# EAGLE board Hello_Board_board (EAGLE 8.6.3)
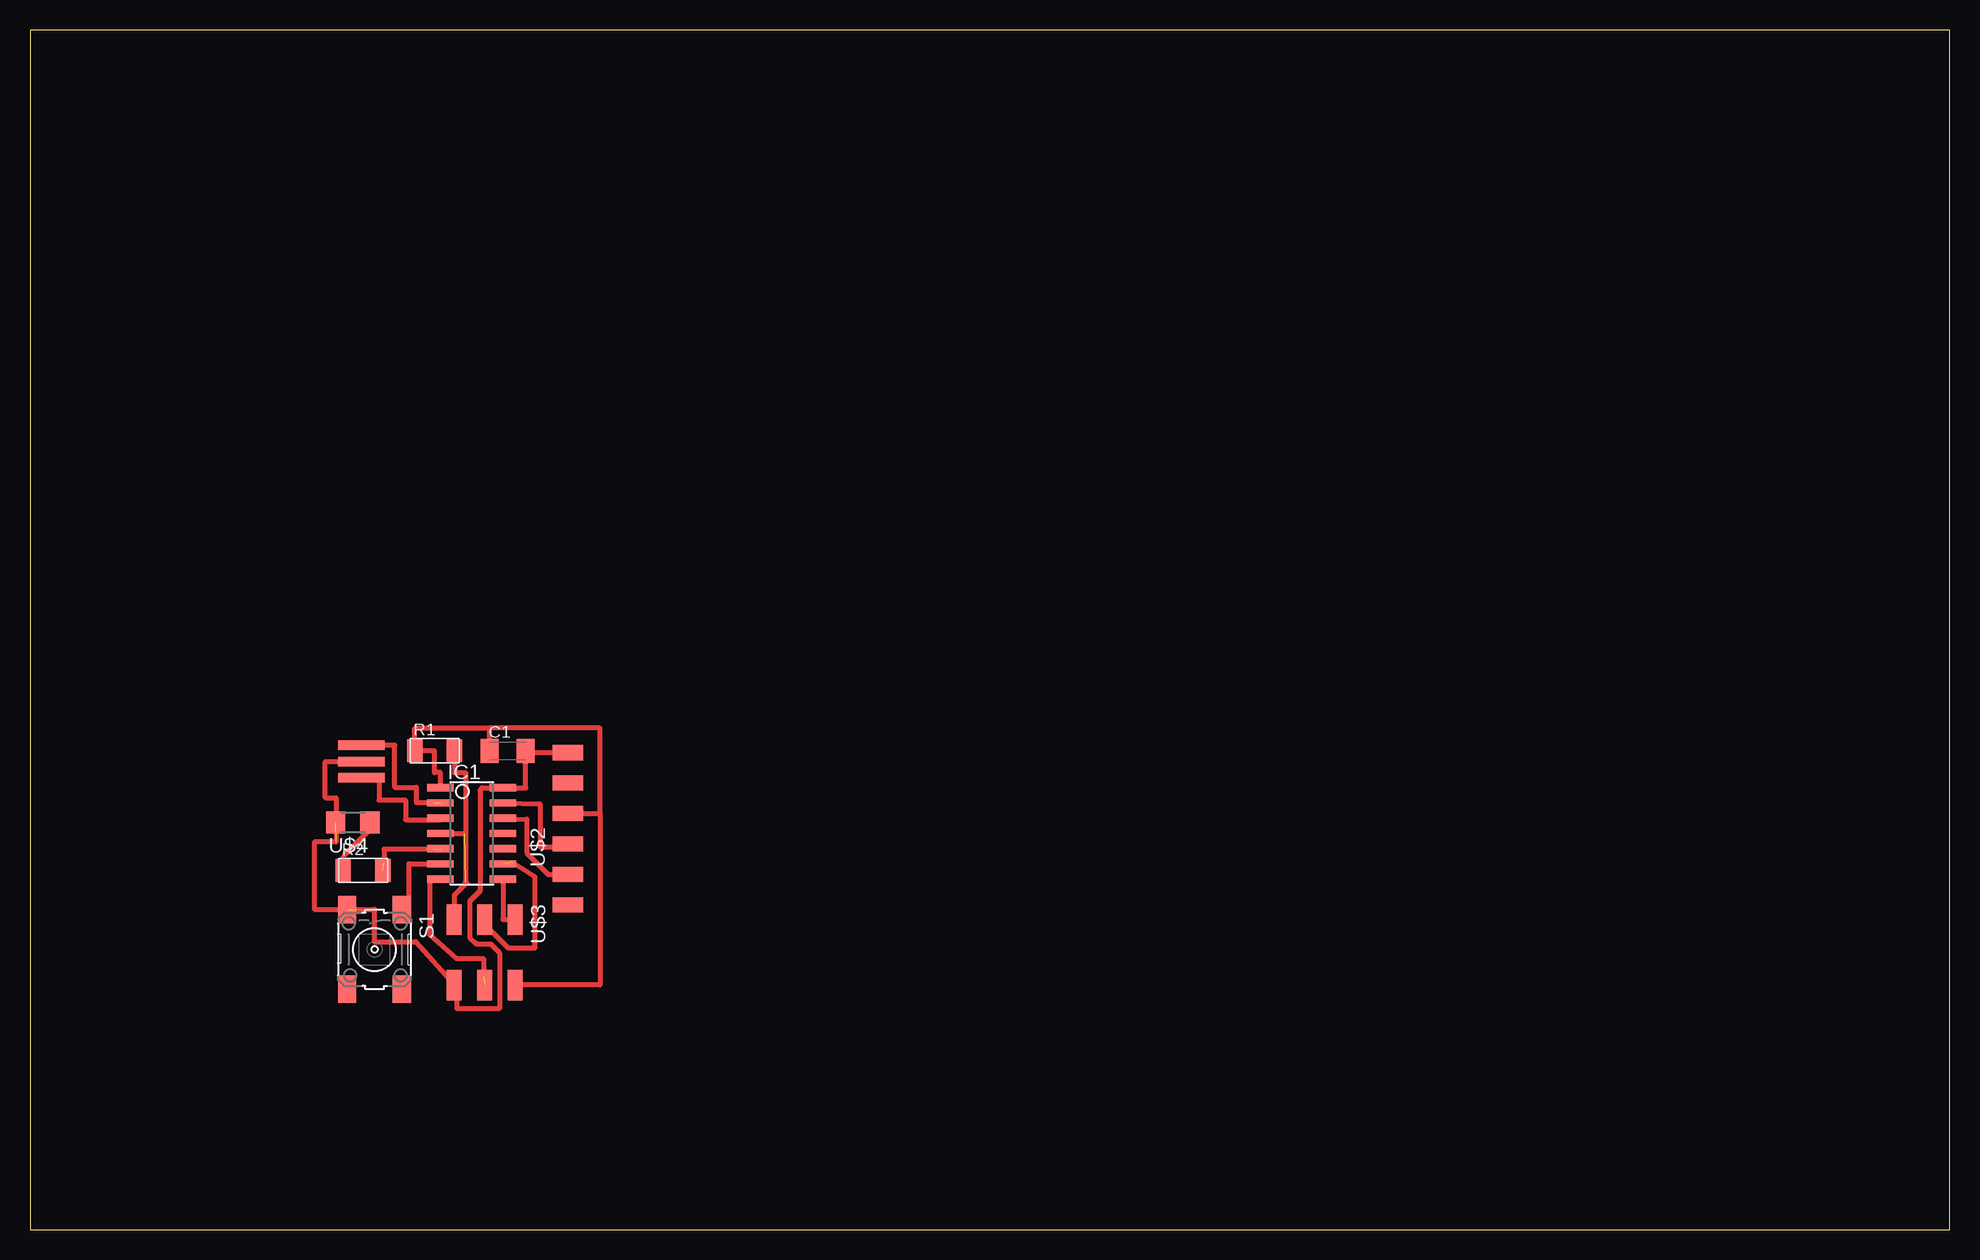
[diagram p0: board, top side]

Size 160 x 100 mm. Coordinates in mm from the lower left corner, seen from the top.
Outline: 0,0 160,0 160,100 0,100 0,0
Copper layers (1*16): Top 0.035mm / dielectric 1.5mm / Bottom 0.035mm
Design rules "default *": minimum track width 16mil, minimum drill 24mm, track to track 16mil, track to pad 16mil, pad to pad 16mil, via to via 16mil, smd to smd 16mil, copper to edge 40mil, drill to drill 6mil, minimum pad ring 10mil, minimum via ring 8mil, stop-mask expansion 4mil, vias tented up to drill 0mil, thermal gap 10mil

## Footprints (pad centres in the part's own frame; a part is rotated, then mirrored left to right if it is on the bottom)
C1206K = smd 1.5 x 2: 1 -1.5,0; 2 1.5,0
SOIC14 = smd 0.61 x 2.21: 1 -3.81,-2.603; 2 -2.54,-2.603; 3 -1.27,-2.603; 4 0,-2.603; 5 1.27,-2.603; 6 2.54,-2.603; 7 3.81,-2.603; 8 3.81,2.603; 9 2.54,2.603; 10 1.27,2.603; 11 0,2.603; 12 -1.27,2.603; 13 -2.54,2.603; 14 -3.81,2.603
R1206FAB = smd 1.27 x 1.905: 1 -1.651,0; 2 1.651,0
6MM_SWITCH = smd 2.286 x 1.524: 1 -3.302,2.286; 2 3.302,2.286; 3 -3.302,-2.286; 4 3.302,-2.286
1X06SMD = smd 2.54 x 1.27: 1 0,6.35; 2 0,3.81; 3 0,1.27; 4 0,-1.27; 5 0,-3.81; 6 0,-6.35
2X03SMD = smd 2.54 x 1.27: 1 -2.54,2.54; 2 2.92,2.54; 3 -2.54,0; 4 2.92,0; 5 -2.54,-2.54; 6 2.92,-2.54
LED1206 = smd 1.6 x 1.803: 1 -1.422,0; 2 1.422,0
EFOBM = smd 0.8 x 3.9: 1 -1.35,0; 2 0,0; 3 1.35,0

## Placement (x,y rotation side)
C1  1 uF  [C1206K]  39.82,39.89 0 top
IC1  ATTINY44-SSU  [SOIC14]  36.83,33.02 270 top
R1  10k  [R1206FAB]  33.73,39.92 0 top
R2  100  [R1206FAB]  27.76,29.94 0 top
S1  [6MM_SWITCH]  28.72,23.35 270 top
U$2  FTDI-SMD-HEADER  [1X06SMD]  44.85,33.41 0 top
U$3  AVRISPSMD  [2X03SMD]  37.9,23.31 270 top
U$4  LED  [LED1206]  26.91,33.94 180 top
XTAL  20 Mhz  [EFOBM]  27.62,39.01 270 top

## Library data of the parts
C1 IC1 R1 R2 S1 U$2-U$4 XTAL = fab

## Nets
N$1: IC1.2 XTAL.1
N$2: IC1.3 XTAL.3
N$3: C1.2 IC1.14 S1.3 U$2.1 U$3.6 U$4.2 XTAL.2
N$4: IC1.4 R1.2 U$3.5
N$5: IC1.5 R2.2
N$6: C1.1 IC1.1 R1.1 U$2.3 U$3.2
N$7: R2.1 U$4.1
N$8: IC1.7 U$3.4
N$9: IC1.9 U$3.3
N$10: IC1.8 U$3.1
N$11: IC1.12 U$2.5
N$12: IC1.13 U$2.4
N$13: IC1.6 S1.1

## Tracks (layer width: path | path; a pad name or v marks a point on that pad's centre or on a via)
N$1  (1 unrouted)
  Top 0.4: 33.7,35.6 32.2,35.6 32.2,36.86 30.4,36.86 30.4,40.36 XTAL.1
N$2
  Top 0.4: IC1.3 34.23,34.16 31.3,34.16 31.3,35.8 29.1,35.8 29.1,37.66 XTAL.3 28.9,37.66
N$3  (2 unrouted)
  Top 0.4: 41.32,36.83 41.32,39.76 | 41.32,36.83 IC1.14 37.7,36.83 37.5,36.63 37.5,28.71 37.5,28.21 36.66,27.37 36.66,24.33 37.01,23.97 37.03,23.97 37.2,23.8 38.4,23.8 39.14,23.06 39.14,18.4 35.6,18.4 35.6,20.39 U$3.6 32.16,24 28.7,24 28.7,26.7 23.7,26.7 23.7,32.3 25.5,32.3 25.5,36 24.61,36 24.61,39.01 XTAL.2 | 41.32,36.83 41.32,36.8 | C1.2 41.32,39.76 | 41.32,39.76 U$2.1
N$4  (1 unrouted)
  Top 0.4: R1.2 35.38,38.1 36.3,38.1 36.3,29 36.4,28.9 35.36,27.86 U$3.5 | IC1.4 36.24,33.02
N$5  (2 unrouted)
  Top 0.4: 29.5,30.6 29.5,31.7 33.6,31.7
N$6
  Top 0.4: U$3.2 47.5,20.39 47.5,34.68 | U$2.3 47.5,34.68 | 47.5,34.68 47.5,41.8 38.32,41.8 | C1.1 38.32,41.8 | 38.32,41.8 32.08,41.8 R1.1 33.7,39.92 33.7,38.1 34.23,38.1 IC1.1
N$7  (1 unrouted)
  Top 0.4: 26.2,31.2 28.33,33.33 U$4.1 | 26.11,31.1 R2.1
N$8  (1 unrouted)
  Top 0.4: 37.8,21.1 37.8,22.6 35.55,22.6 33.3,24.6 | IC1.7 33.3,29.21 | 33.3,29.21 33.3,29.3 | 33.3,29.21 33.3,24.6 | 33.3,24.6 33.4,24.6
N$9  (1 unrouted)
  Top 0.4: U$3.3 37.9,25.44 39.87,23.47 42.1,23.47 42.1,29.4 40.2,30.6
N$10
  Top 0.4: U$3.1 39.43,25.85 IC1.8
N$11
  Top 0.4: IC1.12 41.4,34.2 41.4,31.4 43.2,29.6 U$2.5
N$12
  Top 0.4: U$2.4 44.85,31.9 42.5,31.9 42.5,35.5 IC1.13
N$13
  Top 0.4: S1.1 31.6,26.65 31.6,30.48 IC1.6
